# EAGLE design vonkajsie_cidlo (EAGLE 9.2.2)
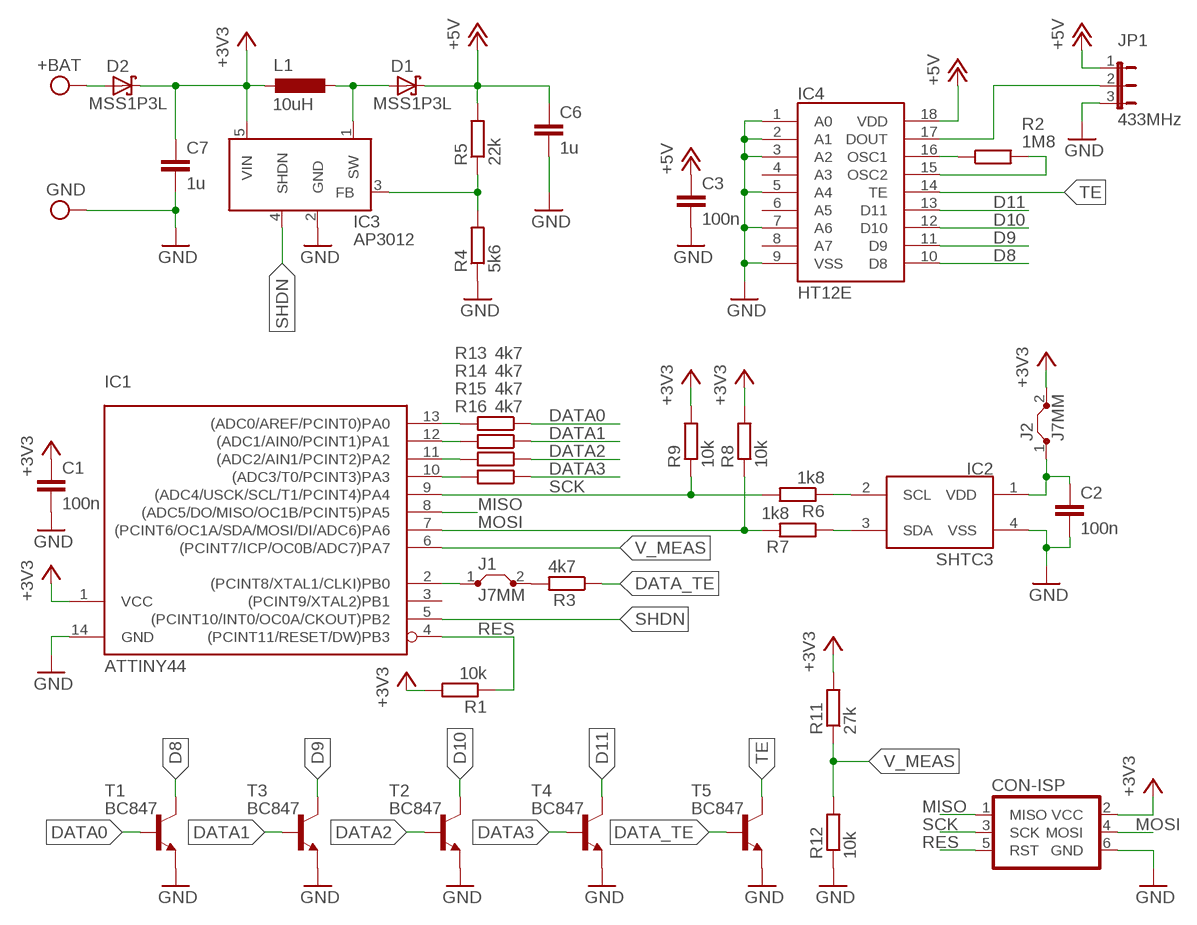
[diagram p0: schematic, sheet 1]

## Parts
C1  100n  C-EUC1206  [C1206]
C2  100n  C-EUC1206  [C1206]
C3  100n  C-EUC1206  [C1206]
C6  1u  C-EUC1206  [C1206]
C7  1u  C-EUC1206  [C1206]
CON-ISP  CON-ISP6  [CON-ISP6]
D1  MSS1P3L  SCHOTKY_2X3  [SCHOTKY_2X3]
D2  MSS1P3L  SCHOTKY_2X3  [SCHOTKY_2X3]
IC1  ATTINY44  [SO14]
IC2  SHTC3  [DFN4]
IC3  AP3012  [SOT23-5]
IC4  HT12E  [DIL18]
J1  J7MM  [07]
J2  J7MM  [07]
JP1  433MHz  JP2E  [JP2]
L1  10uH  L5X5  [L-5X5]
R1  10k  R-EU_R1206  [R1206]
R2  1M8  R-EU_R1206  [R1206]
R3  4k7  R-EU_R0805  [R0805]
R4  5k6  R-EU_R1206  [R1206]
R5  22k  R-EU_R1206  [R1206]
R6  1k8  R-EU_R1206  [R1206]
R7  1k8  R-EU_R1206  [R1206]
R8  10k  R-EU_R1206  [R1206]
R9  10k  R-EU_R1206  [R1206]
R11  27k  R-EU_R1206  [R1206]
R12  10k  R-EU_R0805  [R0805]
R13  4k7  R-EU_R0805  [R0805]
R14  4k7  R-EU_R0805  [R0805]
R15  4k7  R-EU_R0805  [R0805]
R16  4k7  R-EU_R0805  [R0805]
T1  BC847  [SOT23]
T2  BC847  [SOT23]
T3  BC847  [SOT23]
T4  BC847  [SOT23]
T5  BC847  [SOT23]
X1  W237-102  [W237-102]

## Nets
+3V3: C1.1 C7.1 CON-ISP.2(VCC) D2.C IC1.1(VCC) IC3.5(VIN) J2.2 L1.P$1 R1.2 R8.2 R9.2 R11.2
+5V: C3.1 C6.1 D1.C IC4.18(VDD) JP1.1 R5.2
D8: IC4.10(D8) T1.3(C)
D9: IC4.11(D9) T3.3(C)
D10: IC4.12(D10) T2.3(C)
D11: IC4.13(D11) T4.3(C)
DATA0: R13.1 T1.1(B)
DATA1: R14.1 T3.1(B)
DATA2: R15.1 T2.1(B)
DATA3: R16.1 T4.1(B)
DATA_TE: R3.1 T5.1(B)
GND: C1.2 C2.2 C3.2 C6.2 C7.2 CON-ISP.6(GND) IC1.14(GND) IC2.4(VSS) IC3.2(GND) IC4.1(A0) IC4.2(A1) IC4.3(A2) IC4.5(A4) IC4.7(A6) IC4.9(VSS) JP1.3 R4.1 R12.1 T1.2(E) T2.2(E) T3.2(E) T4.2(E) T5.2(E) X1.1
MISO: CON-ISP.1(MISO) IC1.8((ADC5/DO/MISO/OC1B/PCINT5)PA5)
MOSI: CON-ISP.4(MOSI) IC1.7((PCINT6/OC1A/SDA/MOSI/DI/ADC6)PA6) R7.2 R8.1
N$1: IC4.15(OSC2) R2.2
N$2: IC4.16(OSC1) R2.1
N$3: J1.2 R3.2
N$4: IC1.13((ADC0/AREF/PCINT0)PA0) R13.2
N$5: D1.A IC3.1(SW) L1.P$2
N$6: IC1.12((ADC1/AIN0/PCINT1)PA1) R14.2
N$7: IC1.11((ADC2/AIN1/PCINT2)PA2) R15.2
N$8: IC4.17(DOUT) JP1.2
N$9: IC3.3(FB) R4.2 R5.1
N$10: IC2.3(SDA) R7.1
N$11: IC1.10((ADC3/T0/PCINT3)PA3) R16.2
N$12: IC2.2(SCL) R6.1
N$13: IC1.2((PCINT8/XTAL1/CLKI)PB0) J1.1
N$14: C2.1 IC2.1(VDD) J2.1
N$15: D2.A X1.2
RES: CON-ISP.5(RST) IC1.4((PCINT11/RESET/DW)PB3) R1.1
SCK: CON-ISP.3(SCK) IC1.9((ADC4/USCK/SCL/T1/PCINT4)PA4) R6.2 R9.1
SHDN: IC1.5((PCINT10/INT0/OC0A/CKOUT)PB2) IC3.4(SHDN)
TE: IC4.14(TE) T5.3(C)
V_MEAS: IC1.6((PCINT7/ICP/OC0B/ADC7)PA7) R11.1 R12.2
Unconnected: IC1.3((PCINT9/XTAL2)PB1) IC4.4(A3) IC4.6(A5) IC4.8(A7)

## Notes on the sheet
- +BAT
- GND

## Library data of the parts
C1-C3 C6 C7 = rcl:C-EU: CAPACITOR, European symbol
CON-ISP = #Matej:CON-ISP6
D1 D2 = #Matej:SCHOTKY_2X3
IC1 = #Matej:ATTINY44
IC2 = #Matej:SHTC3
IC3 = #Matej:AP3012
IC4 = #Matej:HT12E
J1 J2 = jumper:J: Bridge
JP1 = jumper:JP2E: JUMPER
L1 = #Matej:L5X5
R1-R9 R11-R16 = rcl:R-EU_: RESISTOR, European symbol
T1-T5 = transistor:BC847: NPN TRANSISTOR
X1 = con-wago-500:W237-102: WAGO SCREW CLAMP; MPN: 237-102; OC_FARNELL: unknown; OC_NEWARK: 70K9898

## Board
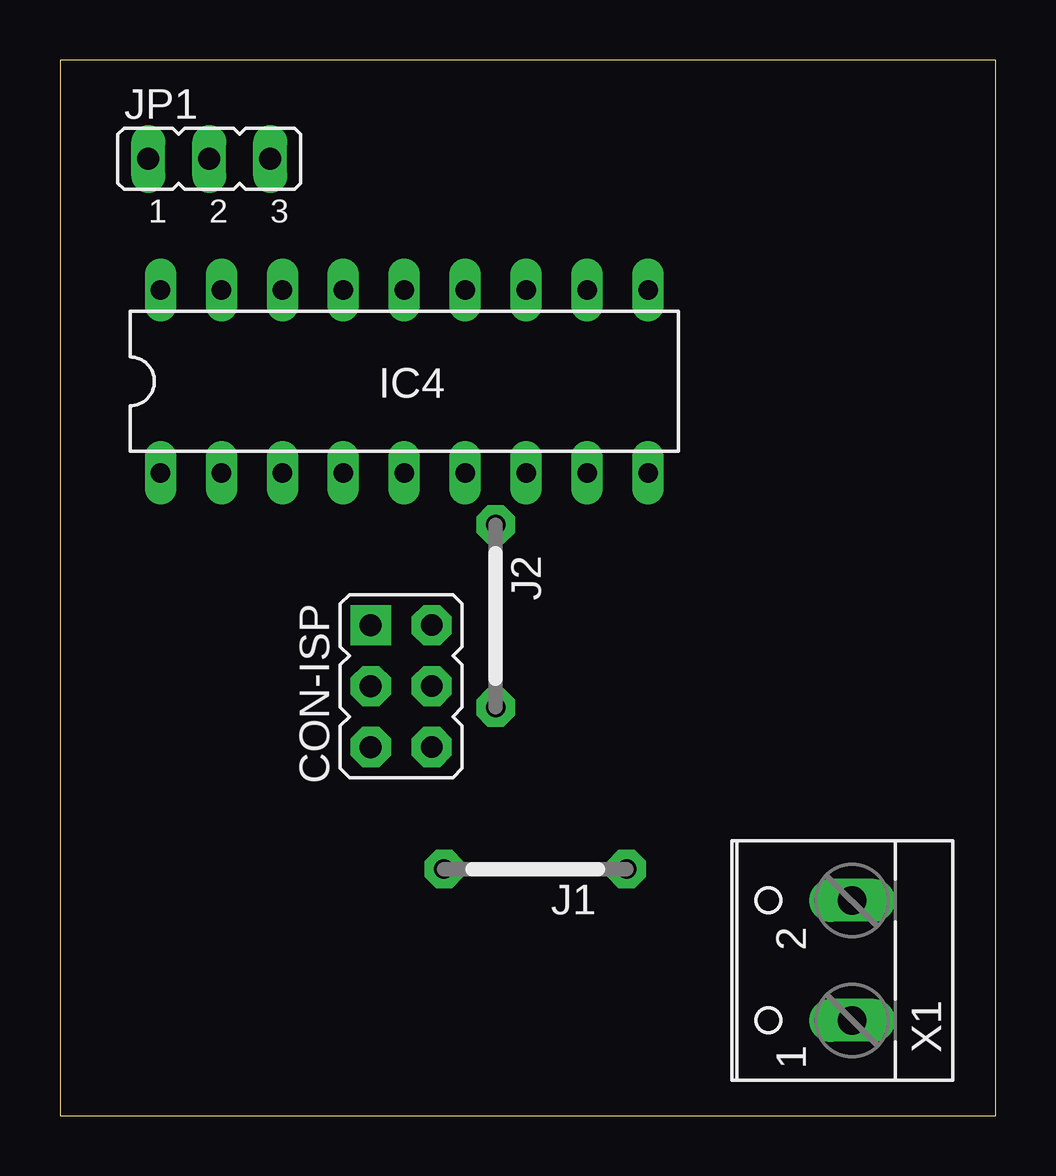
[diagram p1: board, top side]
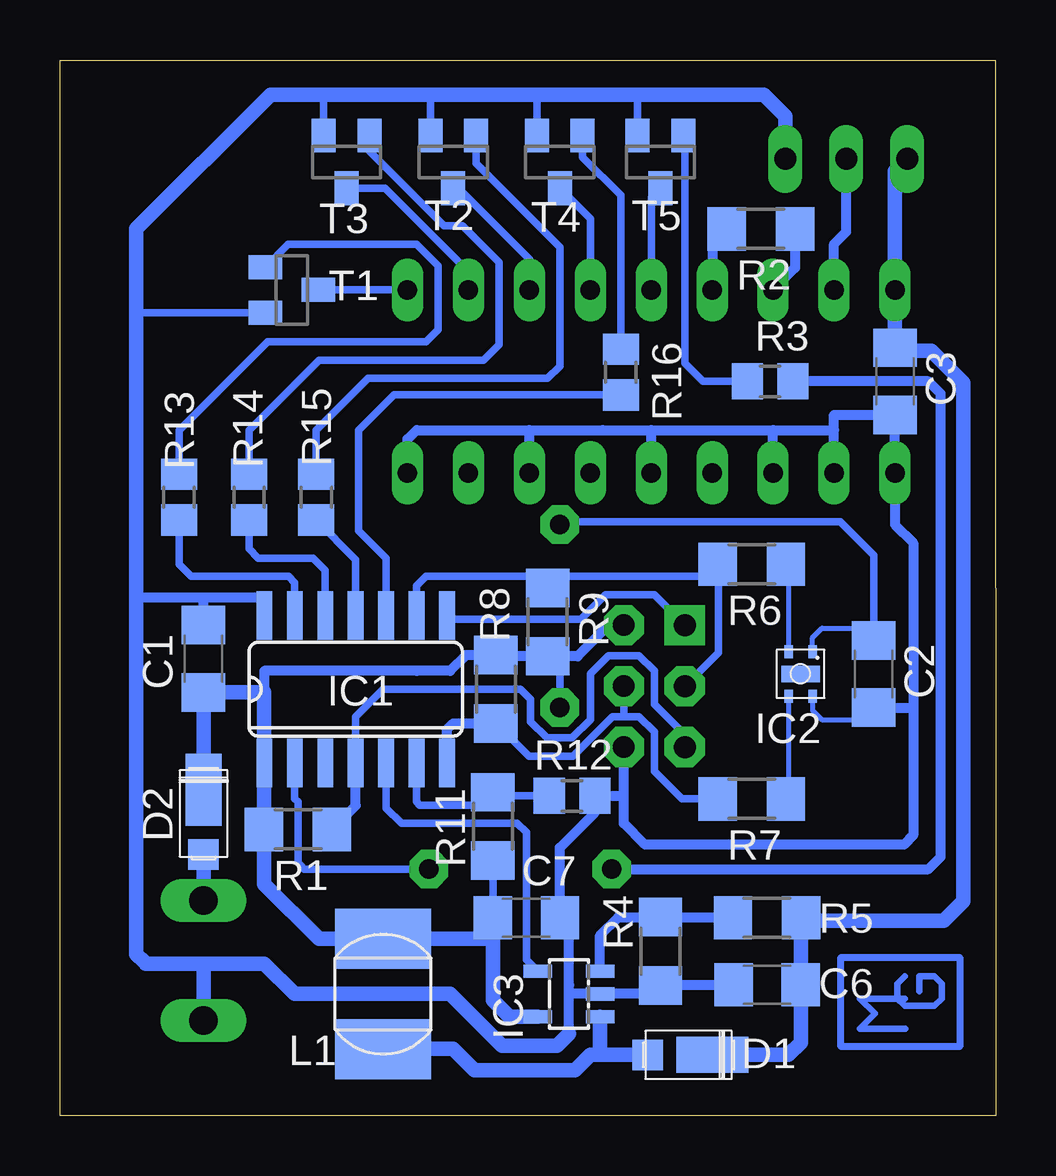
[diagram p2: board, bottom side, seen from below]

Size 39 x 44 mm. Coordinates in mm from the lower left corner, seen from the top.
Outline: 0,0 39,0 39,44 0.01,43.99 0,0
Copper layers (1*16): Top 0.035mm / dielectric 1.5mm / Bottom 0.035mm
Design rules "default *": minimum track width 6mil, minimum drill 0.35mm, track to track 6mil, track to pad 6mil, pad to pad 6mil, via to via 6mil, smd to smd 6mil, copper to edge 40mil, drill to drill 6mil, minimum pad ring 10mil, minimum via ring 8mil, stop-mask expansion 4mil, vias tented up to drill 0mil, thermal gap 10mil

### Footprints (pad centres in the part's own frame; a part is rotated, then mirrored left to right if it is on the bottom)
C1206 = smd 1.6 x 1.8: 1 -1.4,0; 2 1.4,0
CON-ISP6 = drill 0.914 pad 1.676 square: 1 -2.54,-1.27 | drill 0.9 pad 1.676 octagon: 2 -2.54,1.27; 4 0,1.27; 6 2.54,1.27 | drill 0.914 pad 1.676 octagon: 3 0,-1.27; 5 2.54,-1.27
SCHOTKY_2X3 = smd 1.27 x 1.27: A -1.8,0 | smd 3 x 1.5: C 0.9,0
SO14 = smd 0.66 x 2.032: 1 -3.81,-3.073; 2 -2.54,-3.073; 3 -1.27,-3.073; 4 0,-3.073; 5 1.27,-3.073; 6 2.54,-3.073; 7 3.81,-3.073; 8 3.81,3.073; 9 2.54,3.073; 10 1.27,3.073; 11 0,3.073; 12 -1.27,3.073; 13 -2.54,3.073; 14 -3.81,3.073
DFN4 = smd 0.7 x 1.6: 0 0,0 | smd 0.55 x 0.35: 1 -0.925,0.5; 2 -0.925,-0.5; 3 0.925,-0.5; 4 0.925,0.5
SOT23-5 = smd 0.55 x 1.2: 1 -0.95,-1.3; 2 0,-1.3; 3 0.95,-1.3; 4 0.95,1.3; 5 -0.95,1.3
DIL18 = drill 0.813 long: 1 -10.16,-3.81; 2 -7.62,-3.81; 3 -5.08,-3.81; 4 -2.54,-3.81; 5 0,-3.81; 6 2.54,-3.81; 7 5.08,-3.81; 8 7.62,-3.81; 9 10.16,-3.81; 10 10.16,3.81; 11 7.62,3.81; 12 5.08,3.81; 13 2.54,3.81; 14 0,3.81; 15 -2.54,3.81; 16 -5.08,3.81; 17 -7.62,3.81; 18 -10.16,3.81
07 = drill 0.813 pad 1.6 octagon: 1 -3.81,0; 2 3.81,0
JP2 = drill 0.914 long: 1 -2.54,0; 2 0,0; 3 2.54,0
L-5X5 = smd 4 x 2.5: P$1 0,2.3; P$2 0,-2.3
R1206 = smd 1.6 x 1.803: 1 -1.422,0; 2 1.422,0
R0805 = smd 1.3 x 1.5: 1 -0.95,0; 2 0.95,0
SOT23 = smd 1 x 1.4: 1 -0.95,-1.1; 2 0.95,-1.1; 3 0,1.1
W237-102 = drill 1.194 long: 1 -2.5,-1.27; 2 2.5,-1.27

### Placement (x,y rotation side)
C1  33.02,19.05 90 bottom
C2  5.08,18.41 270 bottom
C3  4.19,30.61 270 bottom
C6  9.53,5.46 180 bottom
C7  19.56,8.26 0 bottom
CON-ISP  14.22,17.91 270 top
D1  12.7,2.54 0 bottom
D2  33.02,12.7 90 bottom
IC1  26.67,17.78 0 bottom
IC2  8.13,18.41 270 bottom
IC3  17.78,5.08 90 bottom
IC4  14.35,30.61 0 top
J1  19.81,10.29 180 top
J2  18.16,20.83 270 top
JP1  6.22,39.88 0 top
L1  25.53,5.08 0 bottom
R1  29.08,11.94 180 bottom
R2  9.78,36.96 180 bottom
R3  9.4,30.61 0 bottom
R4  13.97,6.86 90 bottom
R5  9.53,8.26 0 bottom
R6  10.16,22.99 180 bottom
R7  10.16,13.21 180 bottom
R8  20.83,17.78 90 bottom
R9  18.67,20.57 270 bottom
R11  20.95,12.06 270 bottom
R12  17.65,13.34 180 bottom
R13  34.04,25.78 270 bottom
R14  31.11,25.78 270 bottom
R15  28.32,25.78 270 bottom
R16  15.62,30.99 270 bottom
T1  29.34,34.42 270 bottom
T2  22.61,39.75 180 bottom
T3  27.05,39.75 180 bottom
T4  18.16,39.75 180 bottom
T5  13.97,39.75 180 bottom
U$1  [#MG1-VECTOR]  1.27,2.54 90 bottom
X1  31.75,6.48 90 top

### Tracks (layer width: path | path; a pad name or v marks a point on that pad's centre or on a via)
+3V3
  Bottom 0.305: R11.2 C7.1 | J2.2 18.16,19.15
  Bottom 0.406: 30.48,17.65 30.48,18.54 24.13,18.54 22.73,18.54 22.07,19.2 R8.2 20.78,19.15 R9.2 18.16,19.15 17.42,19.15 16.13,20.45 CON-ISP.2 | R1.2 30.33,12.12 30.18,12.12 30.48,12.42 30.48,12.7 | C7.1
  Bottom 0.61: 30.48,12.7 IC1.1 30.48,17.65 C1.1 D2.C | R1.2 30.48,11.91 30.48,9.65 28.21,7.38 L1.P$1 20.97,7.38 20.95,7.37 | 20.95,7.37 20.95,4.83 20.26,4.13 IC3.5 | 20.95,7.37 C7.1
+5V
  Bottom 0.305: C3.1 4.06,31.88
  Bottom 0.406: 8.12,8.23 R5.2 7.98,8.13
  Bottom 0.61: C3.1 IC4.18 4.19,39.37 JP1.1 | 8.12,8.23 C6.1 8.12,3.05 8.63,2.54 D1.C | 7.98,8.13 2.16,8.13 1.33,8.95 1.33,30.54 2.67,31.88 4.06,31.88
D8
  Bottom 0.305: IC4.10 T1.3
D9
  Bottom 0.305: T3.3 25.44,38.65 21.97,35.18 IC4.11
D10
  Bottom 0.305: T2.3 22.39,38.65 19.43,35.69 IC4.12
D11
  Bottom 0.305: T4.3 16.89,37.38 IC4.13
DATA0
  Bottom 0.305: R13.1 34.04,28.57 30.35,32.26 23.75,32.26 23.24,32.77 23.24,35.43 24.13,36.32 29.48,36.32 T1.1
DATA1
  Bottom 0.305: R14.1 31.11,28.57 28.19,31.5 21.34,31.5 20.7,32.13 20.7,35.56 22.23,37.08 22.99,37.08 26.1,40.2 T3.1
DATA2
  Bottom 0.305: T2.1 21.66,39.69 18.16,36.2 18.16,31.24 18.67,30.73 26.16,30.73 28.32,28.57 R15.1
DATA3
  Bottom 0.305: R16.1 15.62,38.35 17.21,39.94 T4.1
DATA_TE
  Bottom 0.305: R3.1 12.19,30.61 12.95,31.37 12.95,40.78 T5.1
GND
  Bottom 0.2: IC2.4 7.63,16.9 7.24,16.51 5.58,16.51 C2.2
  Bottom 0.305: 17.78,7.88 C7.2 | T5.2 14.92,42.48 14.99,42.55 | T4.2 19.11,42.48 19.05,42.55 | T2.2 23.56,42.48 23.5,42.55 | T3.2 28,42.48 27.94,42.55 | T1.2 35.75,33.47 35.81,33.53
  Bottom 0.406: IC4.9 24.51,28.19 24.13,28.57 19.43,28.57 | 19.43,28.57 16.38,28.57 14.35,28.57 | 14.35,28.57 9.27,28.57 | 9.27,28.57 6.73,28.57 | IC4.2 6.73,28.57 | 6.73,28.57 6.73,29.21 C3.2 IC4.1 4.19,24.64 3.43,23.88 3.43,17.02 | IC4.3 9.27,28.57 | IC4.5 14.35,28.57 | IC4.7 19.43,28.57 | IC1.14 30.48,21.59 33.02,21.59 | 17.78,7.88 17.78,5.46 17.78,5.08 | C7.2 18.16,10.48 18.16,11.18 16.7,12.63 R12.1 15.49,13.34 | C6.2 10.95,5.44 R4.1 14.33,5.08 IC3.2 17.78,5.08 | 17.78,3.43 17.78,5.08 | 33.02,21.59 35.81,21.59 | C1.2 33.02,21.59 | C2.2 3.43,17.02 | 15.49,13.34 15.49,12.19 14.61,11.3 3.81,11.3 3.43,11.68 3.43,17.02 | 15.49,13.34 CON-ISP.6
  Bottom 0.61: 17.78,3.43 18.29,2.92 20.57,2.92 22.73,5.08 29.21,5.08 30.48,6.35 33.02,6.35 | JP1.3 8.76,41.66 9.65,42.55 14.99,42.55 19.05,42.55 23.5,42.55 27.94,42.55 30.23,42.55 35.81,36.96 35.81,33.53 35.81,21.59 35.81,17.65 35.81,6.73 35.5,6.41 35.43,6.35 33.02,6.35 | X1.1 33.02,6.35
MISO
  Bottom 0.305: CON-ISP.1 14.03,21.53 | 14.03,21.53 14.22,21.72 | 14.03,21.53 14.22,21.72 | 14.22,21.72 16.26,21.72 17.27,20.7 22.71,20.7 IC1.8
MOSI
  Bottom 0.305: 15.49,16.64 14.86,16.64 14.22,16 14.22,14.35 13.08,13.21 R7.2 | CON-ISP.4 15.49,16.64 | 15.49,16.64 15.97,16.64 17.62,14.99 19.46,14.99 R8.1
  Bottom 0.406: IC1.7 22.86,16.1 22.61,16.36 R8.1
N$1
  Bottom 0.406: R2.2 11.81,36.35 IC4.15
N$2
  Bottom 0.406: R2.1 8.36,35.33 IC4.16
N$3
  Bottom 0.406: J1.2 2.79,10.29 2.29,10.79 2.29,30.1 2.79,30.61 R3.2
N$4
  Bottom 0.305: IC1.13 29.21,22.23 29.46,22.48 33.53,22.48 34.04,22.99 R13.2
N$5
  Bottom 0.406: 25.51,2.79 L1.P$2 | 16.48,2.57 16.51,2.54
  Bottom 0.61: 25.51,2.79 22.61,2.79 21.72,1.91 17.53,1.91 16.89,2.54 16.51,2.54 D1.A | IC3.1 16.48,2.57
N$6
  Bottom 0.305: R14.2 31.11,23.62 30.73,23.24 28.45,23.24 27.94,22.73 IC1.12
N$7
  Bottom 0.305: R15.2 26.67,23.18 IC1.11
N$8
  Bottom 0.406: IC4.17 6.73,36.32 6.22,36.83 JP1.2
N$9
  Bottom 0.406: IC3.3 16.48,7.52 15.72,8.28 R4.2 10.97,8.28 R5.1
N$10
  Bottom 0.2: IC2.3 8.63,13.32 R7.1
N$11
  Bottom 0.305: 24.32,30.04 24.13,30.04 | 24.13,30.04 R16.2 | 24.13,30.04 25.08,30.04 26.54,28.57 26.54,24.38 25.4,23.24 IC1.10
N$12
  Bottom 0.2: R6.1 8.63,22.88 IC2.2
N$13
  Bottom 0.305: J1.1 28.83,10.29 28.96,10.41 | 28.96,10.41 29.08,10.54 | 28.96,10.41 29.08,10.54 | IC1.2 29.21,13.21 29.08,13.08 29.08,10.54
N$14
  Bottom 0.203: IC2.1 7.63,19.93 7.24,20.32 5.08,20.32
  Bottom 0.305: J2.1 18.03,24.77 6.48,24.77 5.08,23.37 5.08,20.32 C2.1
N$15
  Bottom 0.61: X1.2 D2.A
RES
  Bottom 0.305: IC1.4 26.67,16.64 25.53,17.78 19.81,17.78 19.39,17.36 19.39,16.43 18.71,15.75 17.65,15.75 16.89,16.51 16.89,18.41 16.13,19.18 14.86,19.18 14.22,18.54 14.22,17.14 12.95,15.88 CON-ISP.5
  Bottom 0.406: R1.1 26.67,12.93 IC1.4
SCK
  Bottom 0.305: CON-ISP.3 11.56,19.3 11.56,21.59 11.56,22.48 | IC1.9 24.13,22.1 23.75,22.48 18.67,22.48 | 18.67,22.48 12.7,22.48 11.56,22.48 | R9.1 18.67,22.48 | R6.2 11.56,22.99 11.56,22.48
SHDN
  Bottom 0.305: IC3.4 19.56,6.51 19.56,11.81 19.94,12.19 24.77,12.19 25.4,12.83 IC1.5
TE
  Bottom 0.305: T5.3 14.35,38.27 IC4.14
V_MEAS
  Bottom 0.305: R12.2 20.8,13.34 R11.1 21.49,12.95 24,12.95 24.13,13.08 IC1.6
